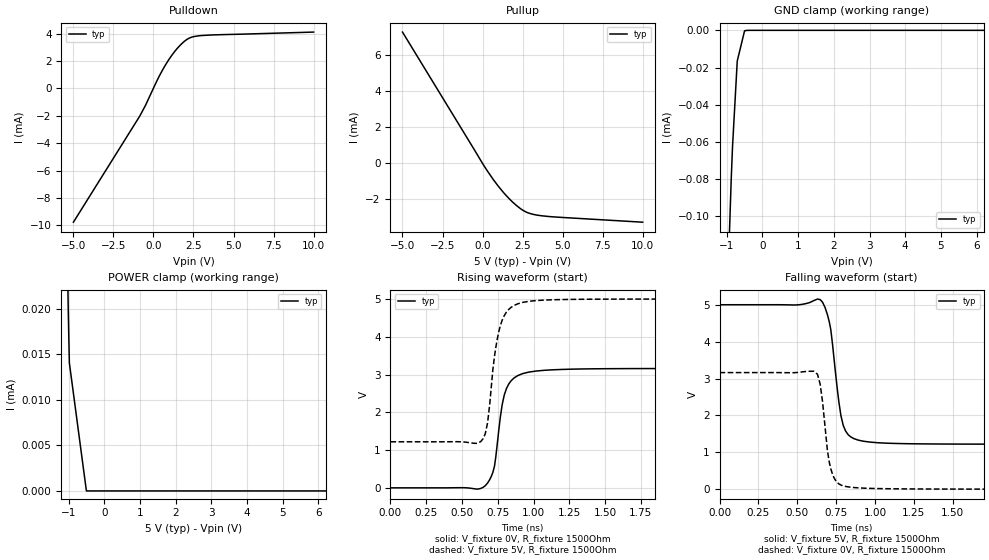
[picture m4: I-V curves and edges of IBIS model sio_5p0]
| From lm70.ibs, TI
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|   sio_5p0 Model
[Model]   sio_5p0
Model_type   3-state
Polarity   Non-Inverting
Vmeas = 2.5
Vref = 0
Cref = 80pF
Rref = 4000
|   typ   min   max
|   (nom PVT)   (fast PVT)   (slow PVT)
C_comp   3.305e-14   3.144e-14   3.329e-14
| Where nom  PVT is Nominal Process, 5V, 27C
|   Fast PVT is Strong Process,  5.5V, -55C
|   Slow PVT is Weak Process,   4.5V, 150C
[Voltage Range]   5   4.5   5.5
|Junction Temperature
[Temperature Range]   27   150   -55
[Pullup Reference]   5   4.5   5.5
[Pulldown Reference]   0   0   0
[Power Clamp Reference]   5   4.5   5.5
[GND Clamp Reference]   0   0   0
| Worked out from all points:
|   slope of the pulldown table from 0 to 0.75 V, typ, clamps not added: 443 ohm
|   slope of the pullup table from 0 to 0.75 V, typ, clamps not added: 762 ohm
|   GND clamp passes 1 mA (typ) near -1.30 V on its own axis
|   POWER clamp passes 1 mA (typ) near -1.30 V on its own axis
|   falling waveform, V_fixture 5V, R_fixture 1500Ohm: 20-80 % time 63.9ps typ, NA min, NA max; typ from 5 V to 1.22 V
|   rising waveform, V_fixture 0V, R_fixture 1500Ohm: 20-80 % time 72.4ps typ, NA min, NA max; typ from 0 V to 3.16 V
|   rising waveform, V_fixture 5V, R_fixture 1500Ohm: 20-80 % time 78ps typ, NA min, NA max; typ from 1.22 V to 5 V
|   falling waveform, V_fixture 0V, R_fixture 1500Ohm: 20-80 % time 53.8ps typ, NA min, NA max; typ from 3.16 V to 0 V
[Pulldown]
|   Voltage   I(typ)   I(min)   I(max)
-5V       -9.768mA   NA         NA
-855mV    -2.022mA   NA         NA
-500mV    -1.247mA   NA         NA
305mV     760.1uA    NA         NA
797mV     1.798mA    NA         NA
1.395V    2.788mA    NA         NA
1.993V    3.488mA    NA         NA
2.385V    3.736mA    NA         NA
3.1V      3.862mA    NA         NA
10V       4.105mA    NA         NA
[GND Clamp]
|   Voltage   I(typ)   I(min)   I(max)
-5V       -96.83mA   NA         NA
-1.084V   -202.2uA   NA         NA
-873.5mV  -80.07uA   NA         NA
-835mV    -61.84uA   NA         NA
-704.5mV  -16.49uA   NA         NA
-500mV    -278.8nA   NA         NA
10V       0A         NA         NA
[Pullup]
|   Voltage   I(typ)   I(min)   I(max)
-5V       7.254mA    NA         NA
302mV     -424.8uA   NA         NA
700mV     -933.1uA   NA         NA
1.3V      -1.606mA   NA         NA
2.123V    -2.336mA   NA         NA
2.5V      -2.586mA   NA         NA
2.826V    -2.734mA   NA         NA
3.699V    -2.902mA   NA         NA
10V       -3.256mA   NA         NA
[POWER Clamp]
|   Voltage   I(typ)   I(min)   I(max)
-5V       112.7mA    NA         NA
-1.103V   45.7uA     NA         NA
-1.012V   20.86uA    NA         NA
-990mV    16.37uA    NA         NA
-977mV    14.07uA    NA         NA
-500mV    0A         NA         NA
10V       0A         NA         NA
[Ramp]
R_load = 1500
|   typ   min   max
dV/dt_r   1.89636/7.24677e-11   NA   NA
dV/dt_f   2.21149/5.46915e-11   NA   NA
[Falling Waveform]
V_fixture = 5V
V_fixture_min = 4.5V
V_fixture_max = 5.5V
R_fixture = 1500Ohm
|   Time   V(typ)   V(min)   V(max)
0s        5V         NA         NA
500.7ps   4.996V     NA         NA
647ps     5.14V      NA         NA
678.8ps   4.925V     NA         NA
715.5ps   4.328V     NA         NA
767.8ps   2.356V     NA         NA
795.6ps   1.729V     NA         NA
826.6ps   1.481V     NA         NA
889.6ps   1.333V     NA         NA
2.968ns   1.219V     NA         NA
[Rising Waveform]
V_fixture = 0V
V_fixture_min = 0V
V_fixture_max = 0V
R_fixture = 1500Ohm
|   Time   V(typ)   V(min)   V(max)
0s        1.434nV    NA         NA
662.5ps   55.75mV    NA         NA
705.8ps   312.7mV    NA         NA
727ps     570.7mV    NA         NA
767.8ps   1.868V     NA         NA
795.6ps   2.46V      NA         NA
842.7ps   2.833V     NA         NA
923.5ps   3.025V     NA         NA
1.316ns   3.147V     NA         NA
2.968ns   3.161V     NA         NA
[Rising Waveform]
V_fixture = 5V
V_fixture_min = 4.5V
V_fixture_max = 5.5V
R_fixture = 1500Ohm
|   Time   V(typ)   V(min)   V(max)
0s        1.219V     NA         NA
630.1ps   1.223V     NA         NA
662.5ps   1.431V     NA         NA
678.8ps   1.723V     NA         NA
727ps     3.481V     NA         NA
767.8ps   4.294V     NA         NA
810.6ps   4.654V     NA         NA
889.6ps   4.874V     NA         NA
1.256ns   4.991V     NA         NA
2.968ns   5V         NA         NA
[Falling Waveform]
V_fixture = 0V
V_fixture_min = 0V
V_fixture_max = 0V
R_fixture = 1500Ohm
|   Time   V(typ)   V(min)   V(max)
0s        3.161V     NA         NA
606.4ps   3.197V     NA         NA
630.1ps   3.116V     NA         NA
647ps     2.849V     NA         NA
662.5ps   2.374V     NA         NA
694ps     1.042V     NA         NA
715.5ps   553.2mV    NA         NA
745.8ps   241.6mV    NA         NA
795.6ps   89.6mV     NA         NA
2.968ns   17.29uV    NA         NA
